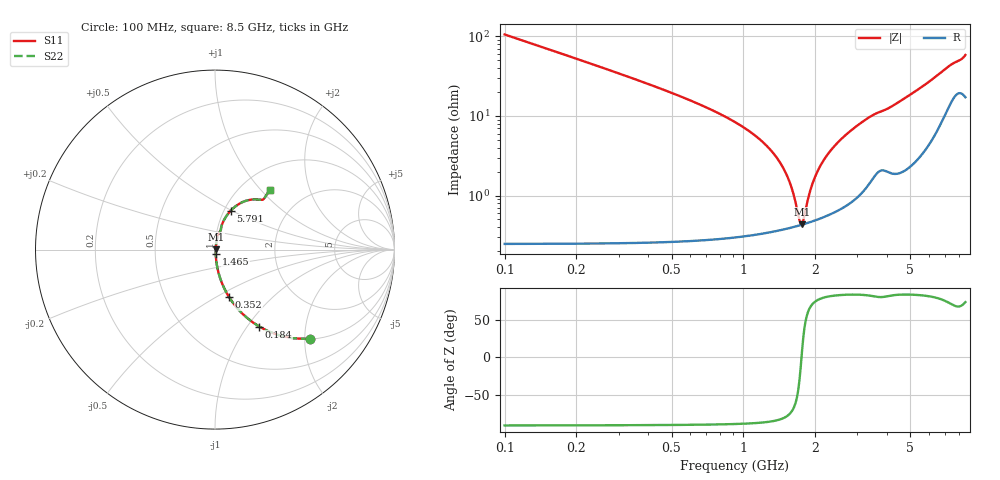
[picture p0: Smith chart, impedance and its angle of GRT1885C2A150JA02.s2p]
!Murata Part Number: GRT1885C2A150JA02
!These Parameters are Measured in Series Mode Connection
!Data Generated on Jun 19, 2026
!  o--ll--o
!Port1  Port2
!  o------o
!Operation Temp=25[degC], DC Bias Voltage=0[V]
!Freq. Start=100[MHz] Stop=9[GHz] 401[Steps]
# Hz S RI R 50
!Freq.(Hz) S11(Real) S11(Imag) S21(Real) S21(Imag) S12(Real) S12(Imag) S22(Real) S22(Imag)
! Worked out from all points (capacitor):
!   401 points, 100 MHz to 8.5 GHz, reference 50 ohm
!   read as one part in series: C = 15 pF near 142 MHz
!   lowest |Z| = 434 mohm at 1.759 GHz (marker M1)
!   series resonance near 1.751 GHz, so ESL is about 550 pH
!   S11 on the Smith chart (normalised r, x): 100 MHz: 1.00, -2.12; 184 MHz: 1.00, -1.14; 352 MHz: 1.01, -0.58; 1.465 GHz: 1.01, -0.04; 5.791 GHz: 1.08, +0.50; 8.5 GHz: 1.34, +1.12
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1e8  0.5279 -0.4981  0.4721 0.4981  0.4721 0.4981  0.5279 -0.4981
1.84e8  0.2465 -0.4288  0.7535 0.4288  0.7535 0.4288  0.2465 -0.4288
2.47e8  0.1522 -0.3562  0.8478 0.3562  0.8478 0.3562  0.1522 -0.3562
3.52e8  0.0793 -0.2659  0.9207 0.2659  0.9207 0.2659  0.0793 -0.2659
6.67e8  0.0209 -0.1333  0.9791 0.1333  0.9791 0.1333  0.0209 -0.1333
1.192e9  0.0056 -0.0479  0.9944 0.0479  0.9944 0.0479  0.0056 -0.0479
1.465e9  0.0042 -0.0219  0.9958 0.0219  0.9958 0.0219  0.0042 -0.0219
1.507e9  0.00413 -0.0185  0.9959 0.0185  0.9959 0.0185  0.00413 -0.0185
1.591e9  0.00408 -0.0118  0.9959 0.0118  0.9959 0.0118  0.00408 -0.0118
1.717e9  0.0042 -0.00239  0.9958 0.00239  0.9958 0.00239  0.0042 -0.00239
1.759e9  0.00428 0.00059  0.9957 -0.00059  0.9957 -0.00059  0.00428 0.00059
1.948e9  0.0049 0.0133  0.9951 -0.0133  0.9951 -0.0133  0.0049 0.0133
2.137e9  0.00586 0.0251  0.9941 -0.0251  0.9941 -0.0251  0.00586 0.0251
2.452e9  0.00819 0.0435  0.9918 -0.0435  0.9918 -0.0435  0.00819 0.0435
2.914e9  0.0135 0.0688  0.9865 -0.0688  0.9865 -0.0688  0.0135 0.0688
3.46e9  0.0251 0.0962  0.9749 -0.0962  0.9749 -0.0962  0.0251 0.0962
4.3e9  0.036 0.1304  0.964 -0.1304  0.964 -0.1304  0.036 0.1304
5.707e9  0.0837 0.2126  0.9163 -0.2126  0.9163 -0.2126  0.0837 0.2126
5.791e9  0.0883 0.2177  0.9117 -0.2177  0.9117 -0.2177  0.0883 0.2177
7.114e9  0.2004 0.2783  0.7996 -0.2783  0.7996 -0.2783  0.2004 0.2783
7.996e9  0.27 0.2808  0.73 -0.2808  0.73 -0.2808  0.27 0.2808
8.5e9  0.3046 0.3317  0.6954 -0.3317  0.6954 -0.3317  0.3046 0.3317
